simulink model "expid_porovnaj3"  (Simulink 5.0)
settings: Solver=ode5  StartTime=0.0  StopTime=500  FixedStep=0.1  RelTol=1e-3

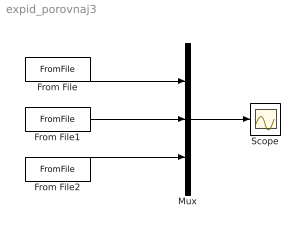
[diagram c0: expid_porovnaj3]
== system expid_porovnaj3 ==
  From File : FromFile  FileName=vstup_u.mat  SampleTime=0
  From File1 : FromFile  FileName=vstup_y.mat  SampleTime=0
  From File2 : FromFile  FileName=vstup_fy.mat  SampleTime=0
  Mux : Mux  Inputs=3
  Scope : Scope
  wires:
  From File1/1 -> Mux/2
  Mux/1 -> Scope/1
  From File/1 -> Mux/1
  From File2/1 -> Mux/3
